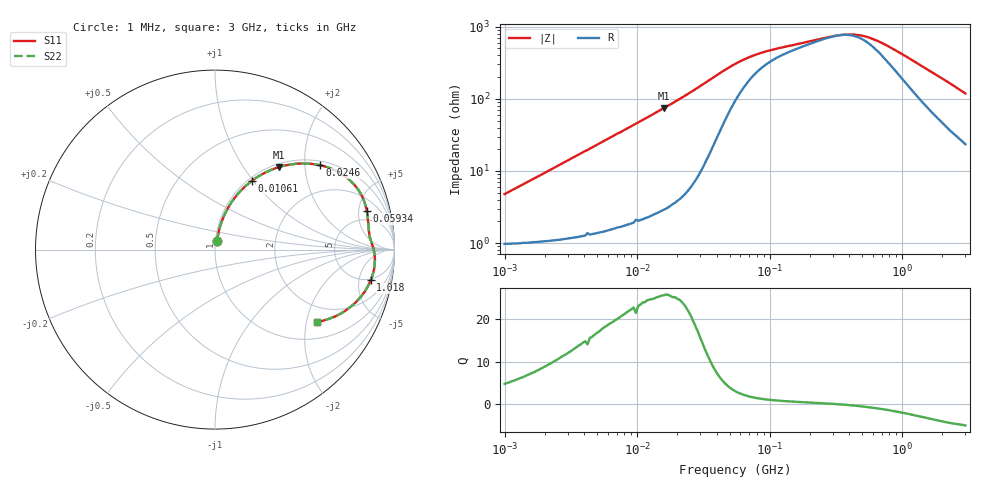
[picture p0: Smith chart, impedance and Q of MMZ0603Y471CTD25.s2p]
! S-parameter Generated by TDK Corporation
! Copyright(C) 2018 TDK Corporation.
! All Rights Reserved.
! TDK P/N: MMZ0603Y471CTD25 (Chip Bead)
! Property: |Z|=470¶ at 100MHz
! Size(LxWxT): 0.6x0.3x0.3mm, 0.024x0.012x0.012inches
! Model Type: s2p (Touchstone File Format Version 1.0)
! Frequency: DC=Yes Start=1MHz Stop=3000MHz 202points Log-sweep
! Model Generated on Aug. 6, 2018
! Port Assignments:
!  1 ---@@@--- 2
! Applicable Conditions:
!  Temperature = 25 degC
!  DC Bias Current = 0 A
!  Small Signal Operation
! Terms and conditions regarding TDK Simulation Models
! (1)This simulation model is being provided solely for informational purposes. Please refer to the specifications of the products in terms of detailed characteristics of such products.
! (2)In no event shall TDK Corporation of any of its subsidiaries be liable for any loss or damage arising, directly or indirectly,
!  From any information contained in this simulation model, including, but not limited to loss or damages arising from any inaccuracies, omissions or errors in connection with such information.
! (3)Any and all copyrights on this simulation model are owned by TDK Corporation.
!  Duplication or redistribution of this simulation model without prior written permission from TDK Corporation is prohibited.
! (4)This simulation model is subject to any modification or change without any prior notice.
! (5)Neither TDK Corporation nor any of its subsidiaries shall make any warranty, express or implied,
!  Including but not limited to the correctness, implied warranties of merchantability and fitness for a particular purpose with respect to this simulation models.
! (6)The use of this simulation model shall be deemed to have consented to the terms and conditions hereof.
# Hz S MA R 50
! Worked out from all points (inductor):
!   201 points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, 1 MHz to 3 GHz, reference 50 ohm
!   read as one part in series: L = 744 nH near 1.041 MHz
!   highest Q = 25.6 at 15.83 MHz (marker M1), where L = 742 nH
!   self-resonance near 337.3 MHz
!   S11 on the Smith chart (normalised r, x): 1 MHz: 1.02, +0.09; 10.61 MHz: 1.04, +0.98; 24.6 MHz: 1.11, +2.38; 59.34 MHz: 3.37, +6.12; 1.018 GHz: 4.65, -7.30; 3 GHz: 1.47, -2.33
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1000000  0.04726 75.6  0.9893 -2.7  0.9893 -2.7  0.04726 75.6
2055611  0.09493 78.2  0.9851 -5.4  0.9851 -5.4  0.09493 78.2
3900413  0.1766 75.9  0.9722 -10.1  0.9722 -10.1  0.1766 75.9
7400828  0.3175 68.7  0.9329 -18.5  0.9329 -18.5  0.3175 68.7
1.061086e7  0.4331 61.9  0.883 -25.6  0.883 -25.6  0.4331 61.9
1.461624e7  0.5517 54.3  0.8125 -33.5  0.8125 -33.5  0.5517 54.3
1.583459e7  0.5834 52.1  0.7897 -35.7  0.7897 -35.7  0.5834 52.1
2.013356e7  0.6765 45.2  0.7096 -42.5  0.7096 -42.5  0.6765 45.2
2.459509e7  0.7492 38.9  0.6286 -48.4  0.6286 -48.4  0.7492 38.9
3.670325e7  0.8509 26.1  0.4425 -57.8  0.4425 -57.8  0.8509 26.1
5.477226e7  0.8738 15.9  0.2877 -56.3  0.2877 -56.3  0.8738 15.9
5.933785e7  0.8727 14.4  0.2659 -54.5  0.2659 -54.5  0.8727 14.4
9.216659e7  0.8647 8.4  0.1921 -41.2  0.1921 -41.2  0.8647 8.4
2.136344e8  0.8719 2.8  0.1357 -18.0  0.1357 -18.0  0.8719 2.8
3.188066e8  0.8827 0.4  0.1175 -2.7  0.1175 -2.7  0.8827 0.4
4.391493e8  0.8898 -2.0  0.1148 15.3  0.1148 15.3  0.8898 -2.0
5.583748e8  0.8932 -4.0  0.1259 30.0  0.1259 30.0  0.8932 -4.0
8.005644e8  0.8917 -7.9  0.1697 46.5  0.1697 46.5  0.8917 -7.9
1.017911e9  0.8841 -11.2  0.2167 52.3  0.2167 52.3  0.8841 -11.2
1.782824e9  0.8305 -21.5  0.3795 53.2  0.3795 53.2  0.8305 -21.5
2.266846e9  0.7828 -27.3  0.471 49.7  0.471 49.7  0.7828 -27.3
3e9  0.6996 -35.3  0.5894 43.3  0.5894 43.3  0.6996 -35.3
